//{{V2}}
ORGANIZATION_BLOCK OB1
TITLE= "Main Program Sweep (Cycle)"


AUTHOR:nb
FAMILY:nb
NAME:nb
VERSION:00.01


VAR_TEMP
       OB1_EV_CLASS:BYTE //Bits 0-3 = 1 (Coming event), Bits 4-7 = 1 (Event class 1)
       OB1_SCAN_1:BYTE //1 (Cold restart scan 1 of OB 1), 3 (Scan 2-n of OB 1)
       OB1_PRIORITY:BYTE //Priority of OB Execution
       OB1_OB_NUMBR:BYTE //1 (Organization block 1, OB1)
       OB1_RESERVED_1:BYTE //Reserved for system
       OB1_RESERVED_2:BYTE //Reserved for system
       OB1_PREV_CYCLE:INT //Cycle time of previous OB1 scan (milliseconds)
       OB1_MIN_CYCLE:INT //Minimum cycle time of OB1 (milliseconds)
       OB1_MAX_CYCLE:INT //Maximum cycle time of OB1 (milliseconds)
       OB1_DATE_TIME:DATE_AND_TIME //Date and time OB1 started
END_VAR
BEGIN

NETWORK
TITLE= Reset
//{{k}}
//Detect when Factory I/O starts running, reset state
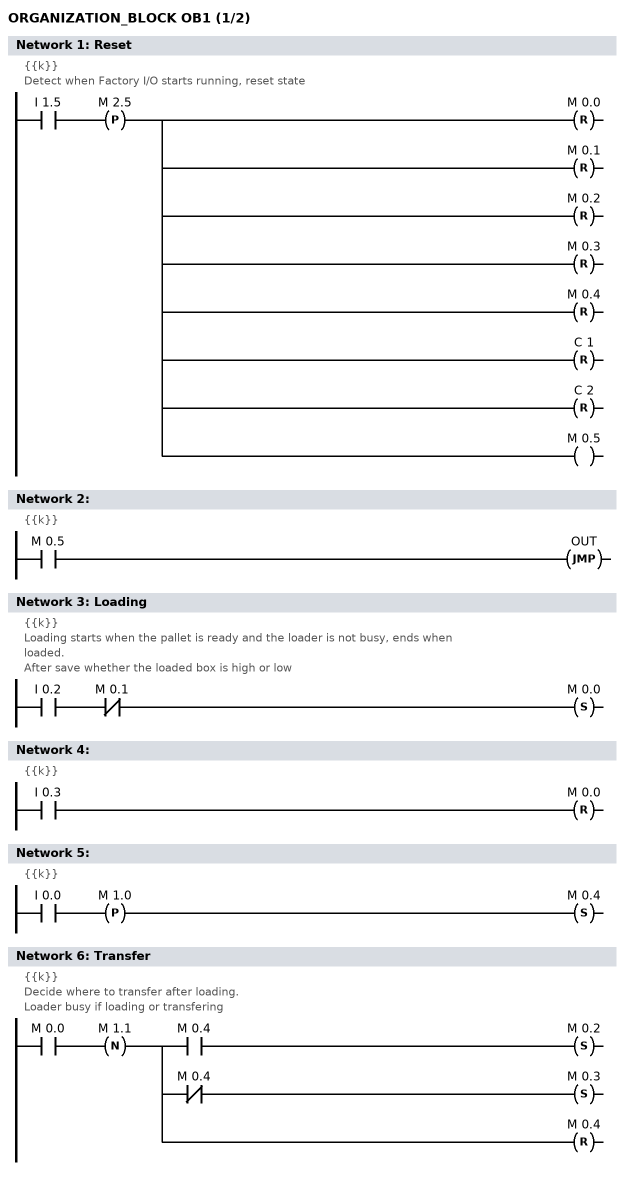
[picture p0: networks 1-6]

       A    I         1.5
       FP   M         2.5
       R    M         0.0
       R    M         0.1
       R    M         0.2
       R    M         0.3
       R    M         0.4
       R    C         1
       R    C         2
       =    M         0.5
NETWORK
TITLE=
//{{k}}
//

       A    M         0.5
       JC   OUT
NETWORK
TITLE= Loading
//{{k}}
//Loading starts when the pallet is ready and the loader is not busy, ends when
//loaded.
//After save whether the loaded box is high or low
//

       A    I         0.2
       AN   M         0.1
       S    M         0.0
NETWORK
TITLE=
//{{k}}
//

       A    I         0.3
       R    M         0.0
NETWORK
TITLE=
//{{k}}
//

       A    I         0.0
       FP   M         1.0
       S    M         0.4
NETWORK
TITLE= Transfer
//{{k}}
//Decide where to transfer after loading.
//Loader busy if loading or transfering

       A    M         0.0
       FN   M         1.1
       =    L        20.0
       A    L        20.0
       A    M         0.4
       S    M         0.2
       A    L        20.0
       AN   M         0.4
       S    M         0.3
       A    L        20.0
       BLD          102
       R    M         0.4
NETWORK
TITLE=
//{{k}}
//
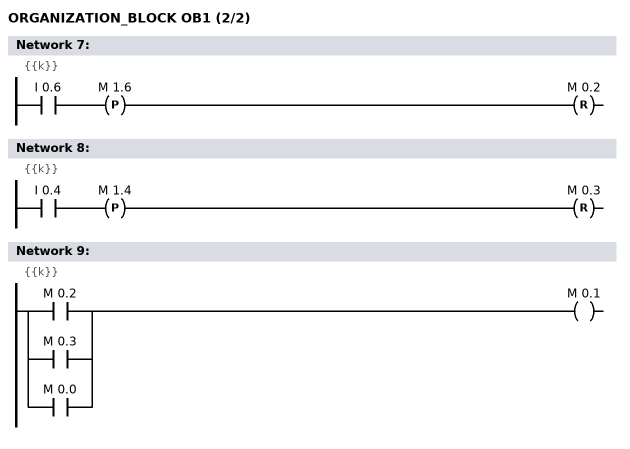
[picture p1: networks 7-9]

       A    I         0.6
       FP   M         1.6
       R    M         0.2
NETWORK
TITLE=
//{{k}}
//

       A    I         0.4
       FP   M         1.4
       R    M         0.3
NETWORK
TITLE=
//{{k}}
//

       O    M         0.2
       O    M         0.3
       O    M         0.0
       =    M         0.1
NETWORK
TITLE= Right Conveyor
//{{k}}
//Increment number of boxes when starting the transfer
//Decrement when exiting

       A    M         0.2
       CU   C         1
       A    I         0.7
       FP   M         1.7
       A    M         3.0
       CD   C         1
       A    M         2.6
       L    C#4
       S    C         1
       A    M         0.5
       R    C         1
       NOP  0
       NOP  0
       A    C         1
       =    M         3.0
NETWORK
TITLE=
//{{k}}
//

       L    MW        3
       BTI
       T    MW        5
       NOP  0
NETWORK
TITLE=
//{{k}}
//

       A    M         0.3
       CU   C         2
       A    I         0.5
       FP   M         1.5
       A    M         3.1
       CD   C         2
       A    M         2.6
       L    C#4
       S    C         2
       A    M         0.5
       R    C         2
       NOP  0
       NOP  0
       A    C         2
       =    M         3.1
NETWORK
TITLE=
//{{k}}
//

       L    MW        4
       BTI
       T    MW        6
       NOP  0
NETWORK
TITLE= Set the ouputs
//{{k}}
//
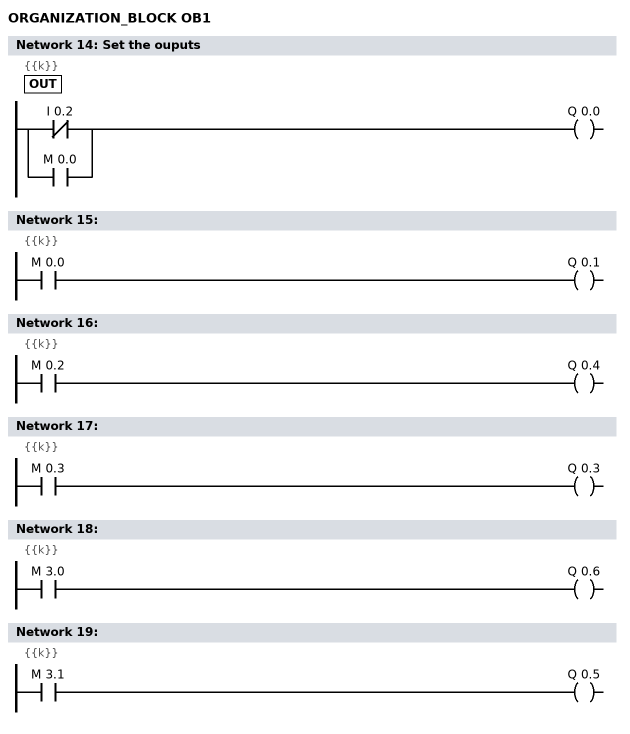
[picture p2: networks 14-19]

OUT   :ON   I         0.2
       O    M         0.0
       =    Q         0.0
NETWORK
TITLE=
//{{k}}
//

       A    M         0.0
       =    Q         0.1
NETWORK
TITLE=
//{{k}}
//

       A    M         0.2
       =    Q         0.4
NETWORK
TITLE=
//{{k}}
//

       A    M         0.3
       =    Q         0.3
NETWORK
TITLE=
//{{k}}
//

       A    M         3.0
       =    Q         0.6
NETWORK
TITLE=
//{{k}}
//

       A    M         3.1
       =    Q         0.5
END_ORGANIZATION_BLOCK
